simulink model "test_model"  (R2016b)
settings: Solver=VariableStepAuto  StartTime=0.0  StopTime=runtime  RelTol=1e-3
InitFcn:
  | clear mex
  | delete test_model_sfun.mexw64
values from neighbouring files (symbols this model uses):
  Delta_T = cell(1,4)    [modelParameters.m]
  F_D = 0    [modelParameters.m]
  g = 9.81    [modelParameters.m]
  Gamma_H = cell(1,4)    [modelParameters.m]
  have_motor_transient = 1    [modelParameters.m]
  height_controlled_o = (((Rm*If        + (((omega0_o * 2 * Rm * Kv * Kq      * Kd + 1)^2) - 1)/(4* Rm*Kv^2*Kq      * Kd))/Vb)*(Pmax - Pmin) + Pmin)    [modelParameters.m]
  i_0 = cell(1,4)    [modelParameters.m]
  If = 0.3836    [modelParameters.m]
  J = diag([ 0.0130 0.0140 0.0285 ])    [modelParameters.m]
  J_L = m_L/12*diag([y_L^2+z_L^2,x_L^2+z_L^2,x_L^2+y_L^2])    [modelParameters.m]
  J_r = cell(1,4)    [modelParameters.m]
  Jreq = 4.2012e-05    [modelParameters.m]
  Jxx = 0.0130    (= 0.013)    [modelParameters.m]
  Jyy = 0.0140    (= 0.014)    [modelParameters.m]
  Jzz = 0.0285    [modelParameters.m]
  K_d = cell(1,4)    [modelParameters.m]
  K_E = cell(1,4)    [modelParameters.m]
  K_H = cell(1,4)    [modelParameters.m]
  K_Q = cell(1,4)    [modelParameters.m]
  K_T = cell(1,4)    [modelParameters.m]
  K_V = cell(1,4)    [modelParameters.m]
  Kd = 1.4852e-07    [modelParameters.m]
  Ki_mahony = 0.001    [modelParameters.m]
  Kp_mahony = 0.4    [modelParameters.m]
  Kq = 96.3422    [modelParameters.m]
  Kt = 1.2007e-05    [modelParameters.m]
  Kv = 96.3422    [modelParameters.m]
  m = 1.216    [modelParameters.m]
  m_L = 0    [modelParameters.m]
  omega0_o = sqrt((m*g)/(4*Kt))    [modelParameters.m]
  omega1_o = sqrt((m*g)/(4*Kt))    [modelParameters.m]
  omega2_o = sqrt((m*g)/(4*Kt))    [modelParameters.m]
  omega3_o = sqrt((m*g)/(4*Kt))    [modelParameters.m]
  omega_0 = cell(1,4)    [modelParameters.m]
  p0 = 0    [modelParameters.m]
  p_0 = cell(1,4)    [modelParameters.m]
  p_max = cell(1,4)    [modelParameters.m]
  phi0 = 0    [modelParameters.m]
  pitch_o = 0    [modelParameters.m]
  pitchrate_o = 0    [modelParameters.m]
  Pmax = 1    [modelParameters.m]
  Pmin = 0    [modelParameters.m]
  psi0 = 0    [modelParameters.m]
  q0 = 0    [modelParameters.m]
  Q_D = 0    [modelParameters.m]
  r0 = 0    [modelParameters.m]
  R_m = cell(1,4)    [modelParameters.m]
  r_oc = [ 0 ; 0 ; 0 ]    [modelParameters.m]
  r_oL = [0; 0; 0]    [modelParameters.m]
  rhx = 0.16    [modelParameters.m]
  rhy = 0.16    [modelParameters.m]
  rhz = 0.03    [modelParameters.m]
  Rm = 0.235    [modelParameters.m]
  roll_o = 0    [modelParameters.m]
  rollrate_o = 0    [modelParameters.m]
  Tc = 0.04    [modelParameters.m]
  theta0 = 0    [modelParameters.m]
  Tq = 0.005    [modelParameters.m]
  u0 = 0    [modelParameters.m]
  v0 = 0    [modelParameters.m]
  Vb = 11.4    [modelParameters.m]
  w0 = 0    [modelParameters.m]
  x0 = 0    [modelParameters.m]
  x_controlled_o = 0    [modelParameters.m]
  x_o = 0    [modelParameters.m]
  x_vel_o = 0    [modelParameters.m]
  y0 = 0    [modelParameters.m]
  y_controlled_o = 0    [modelParameters.m]
  y_o = 0    [modelParameters.m]
  y_vel_o = 0    [modelParameters.m]
  yaw_controlled_o = 0    [modelParameters.m]
  yaw_o = 0    [modelParameters.m]
  yawrate_o = 0    [modelParameters.m]
  z0 = 0    [modelParameters.m]
  z_o = 0    [modelParameters.m]
  z_vel_o = 0    [modelParameters.m]
undefined symbols (not defined in the file or in its folder): Gamma_Omega, Gamma_T, Ki, Kp, r_h, slope, start, Ts, X0
libraries: simulink x16, Derivative x13, dsparch4 x3, vrlib x2
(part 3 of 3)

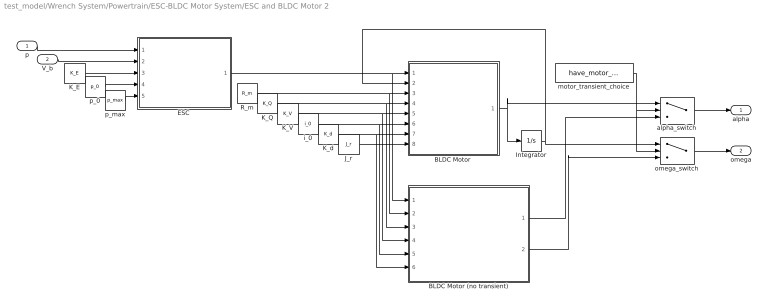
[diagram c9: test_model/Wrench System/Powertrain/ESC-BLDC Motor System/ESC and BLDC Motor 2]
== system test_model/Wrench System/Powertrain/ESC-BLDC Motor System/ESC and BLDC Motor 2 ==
  p : Inport
  V_b : Inport  Port=2
  "BLDC Motor " : MATLAB Function  TreatAsAtomicUnit=on
  BLDC Motor (no transient) : MATLAB Function  TreatAsAtomicUnit=on
  "ESC " : MATLAB Function  TreatAsAtomicUnit=on
  Integrator : Integrator  InitialCondition=omega_0  ContinuousStateAttributes='omega'
  J_r : Constant  Value=J_r
  K_E : Constant  Value=K_E
  K_Q : Constant  Value=K_Q
  K_V : Constant  Value=K_V
  K_d : Constant  Value=K_d
  R_m : Constant  Value=R_m
  alpha_switch : Switch  Criteria=u2 ~= 0
  i_0 : Constant  Value=i_0
  motor_transient_choice : Constant  Value=have_motor_transient
  omega_switch : Switch  Criteria=u2 ~= 0
  p_0 : Constant  Value=p_0
  p_max : Constant  Value=p_max
  alpha : Outport
  omega : Outport  Port=2
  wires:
  motor_transient_choice/1 -> omega_switch/2, alpha_switch/2
  omega_switch/1 -> omega/1
  alpha_switch/1 -> alpha/1
  BLDC Motor (no transient)/2(omega) -> omega_switch/3
  BLDC Motor (no transient)/1(alpha) -> alpha_switch/3
  Integrator/1 -> omega_switch/1, "BLDC Motor "/2(omega)
  "ESC "/1(V) -> BLDC Motor (no transient)/1(V), "BLDC Motor "/1(V)
  p/1 -> "ESC "/1(p)
  V_b/1 -> "ESC "/2(V_b)
  K_E/1 -> "ESC "/3(K_E)
  p_0/1 -> "ESC "/4(p_0)
  p_max/1 -> "ESC "/5(p_max)
  J_r/1 -> "BLDC Motor "/8(J_r)
  R_m/1 -> BLDC Motor (no transient)/2(R_m), "BLDC Motor "/3(R_m)
  "BLDC Motor "/1(alpha) -> alpha_switch/1, Integrator/1
  K_Q/1 -> BLDC Motor (no transient)/3(K_Q), "BLDC Motor "/4(K_Q)
  K_V/1 -> BLDC Motor (no transient)/4(K_V), "BLDC Motor "/5(K_V)
  i_0/1 -> BLDC Motor (no transient)/5(i_0), "BLDC Motor "/6(i_0)
  K_d/1 -> BLDC Motor (no transient)/6(K_d), "BLDC Motor "/7(K_d)

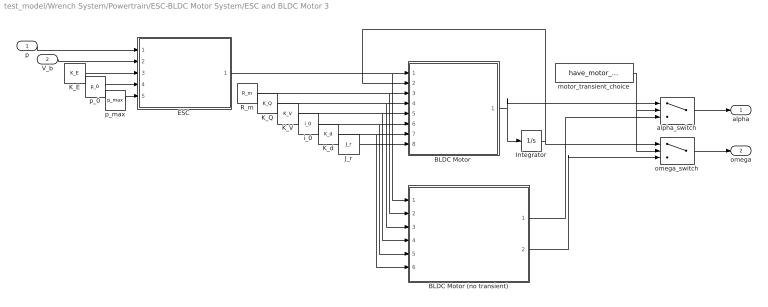
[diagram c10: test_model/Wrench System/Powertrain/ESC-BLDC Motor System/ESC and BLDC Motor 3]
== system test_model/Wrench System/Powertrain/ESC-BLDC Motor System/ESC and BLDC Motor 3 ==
  p : Inport
  V_b : Inport  Port=2
  "BLDC Motor " : MATLAB Function  TreatAsAtomicUnit=on
  BLDC Motor (no transient) : MATLAB Function  TreatAsAtomicUnit=on
  "ESC " : MATLAB Function  TreatAsAtomicUnit=on
  Integrator : Integrator  InitialCondition=omega_0  ContinuousStateAttributes='omega'
  J_r : Constant  Value=J_r
  K_E : Constant  Value=K_E
  K_Q : Constant  Value=K_Q
  K_V : Constant  Value=K_V
  K_d : Constant  Value=K_d
  R_m : Constant  Value=R_m
  alpha_switch : Switch  Criteria=u2 ~= 0
  i_0 : Constant  Value=i_0
  motor_transient_choice : Constant  Value=have_motor_transient
  omega_switch : Switch  Criteria=u2 ~= 0
  p_0 : Constant  Value=p_0
  p_max : Constant  Value=p_max
  alpha : Outport
  omega : Outport  Port=2
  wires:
  motor_transient_choice/1 -> omega_switch/2, alpha_switch/2
  omega_switch/1 -> omega/1
  alpha_switch/1 -> alpha/1
  BLDC Motor (no transient)/2(omega) -> omega_switch/3
  BLDC Motor (no transient)/1(alpha) -> alpha_switch/3
  Integrator/1 -> omega_switch/1, "BLDC Motor "/2(omega)
  "ESC "/1(V) -> BLDC Motor (no transient)/1(V), "BLDC Motor "/1(V)
  p/1 -> "ESC "/1(p)
  V_b/1 -> "ESC "/2(V_b)
  K_E/1 -> "ESC "/3(K_E)
  p_0/1 -> "ESC "/4(p_0)
  p_max/1 -> "ESC "/5(p_max)
  J_r/1 -> "BLDC Motor "/8(J_r)
  R_m/1 -> BLDC Motor (no transient)/2(R_m), "BLDC Motor "/3(R_m)
  "BLDC Motor "/1(alpha) -> alpha_switch/1, Integrator/1
  K_Q/1 -> BLDC Motor (no transient)/3(K_Q), "BLDC Motor "/4(K_Q)
  K_V/1 -> BLDC Motor (no transient)/4(K_V), "BLDC Motor "/5(K_V)
  i_0/1 -> BLDC Motor (no transient)/5(i_0), "BLDC Motor "/6(i_0)
  K_d/1 -> BLDC Motor (no transient)/6(K_d), "BLDC Motor "/7(K_d)

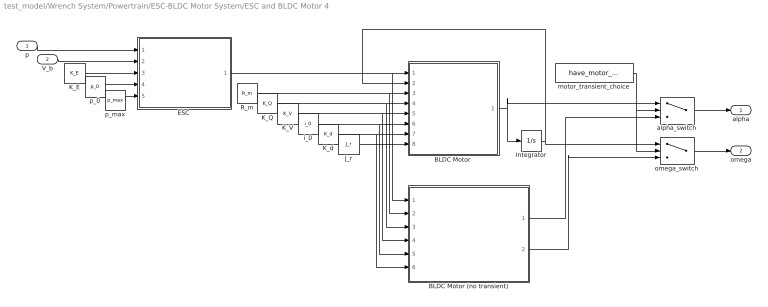
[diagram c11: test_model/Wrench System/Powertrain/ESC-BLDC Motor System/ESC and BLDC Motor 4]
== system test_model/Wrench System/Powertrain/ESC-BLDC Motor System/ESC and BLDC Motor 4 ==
  p : Inport
  V_b : Inport  Port=2
  "BLDC Motor " : MATLAB Function  TreatAsAtomicUnit=on
  BLDC Motor (no transient) : MATLAB Function  TreatAsAtomicUnit=on
  "ESC " : MATLAB Function  TreatAsAtomicUnit=on
  Integrator : Integrator  InitialCondition=omega_0  ContinuousStateAttributes='omega'
  J_r : Constant  Value=J_r
  K_E : Constant  Value=K_E
  K_Q : Constant  Value=K_Q
  K_V : Constant  Value=K_V
  K_d : Constant  Value=K_d
  R_m : Constant  Value=R_m
  alpha_switch : Switch  Criteria=u2 ~= 0
  i_0 : Constant  Value=i_0
  motor_transient_choice : Constant  Value=have_motor_transient
  omega_switch : Switch  Criteria=u2 ~= 0
  p_0 : Constant  Value=p_0
  p_max : Constant  Value=p_max
  alpha : Outport
  omega : Outport  Port=2
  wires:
  motor_transient_choice/1 -> omega_switch/2, alpha_switch/2
  omega_switch/1 -> omega/1
  alpha_switch/1 -> alpha/1
  BLDC Motor (no transient)/2(omega) -> omega_switch/3
  BLDC Motor (no transient)/1(alpha) -> alpha_switch/3
  Integrator/1 -> omega_switch/1, "BLDC Motor "/2(omega)
  "ESC "/1(V) -> BLDC Motor (no transient)/1(V), "BLDC Motor "/1(V)
  p/1 -> "ESC "/1(p)
  V_b/1 -> "ESC "/2(V_b)
  K_E/1 -> "ESC "/3(K_E)
  p_0/1 -> "ESC "/4(p_0)
  p_max/1 -> "ESC "/5(p_max)
  J_r/1 -> "BLDC Motor "/8(J_r)
  R_m/1 -> BLDC Motor (no transient)/2(R_m), "BLDC Motor "/3(R_m)
  "BLDC Motor "/1(alpha) -> alpha_switch/1, Integrator/1
  K_Q/1 -> BLDC Motor (no transient)/3(K_Q), "BLDC Motor "/4(K_Q)
  K_V/1 -> BLDC Motor (no transient)/4(K_V), "BLDC Motor "/5(K_V)
  i_0/1 -> BLDC Motor (no transient)/5(i_0), "BLDC Motor "/6(i_0)
  K_d/1 -> BLDC Motor (no transient)/6(K_d), "BLDC Motor "/7(K_d)

== matlab function test_model/Actuation/Gravity

 ==
function E_Fg = gravity(m, g)

E_Fg = [0; 0; m*g];

== matlab function test_model/Actuation/Lbe





 ==
function E_ro  = linear_body_earth_conversion(B_vo, euler_angles)

euler_rates = zeros(3,1);
E_ro = zeros(3,1);

phi = euler_angles(1);
theta = euler_angles(2);
psi = euler_angles(3);

Leb = [cos(theta)*cos(psi), sin(phi)*sin(theta)*cos(psi)-cos(phi)*sin(psi), cos(phi)*sin(theta)*cos(psi)+sin(phi)*sin(psi); ...
       cos(theta)*sin(psi), sin(phi)*sin(theta)*sin(psi)+cos(phi)*cos(psi), cos(phi)*sin(theta)*sin(psi)-sin(phi)*cos(psi); ...
           -sin(theta)    ,                sin(phi)*cos(theta)            ,                 cos(phi)*cos(theta)           ];

E_ro = Leb * B_vo;

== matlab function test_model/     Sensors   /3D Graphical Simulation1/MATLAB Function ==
function y = eigenaxis_ucart(u)


if abs(u(1))< 0.0001
    u(1) = 0.0001;
end

if abs(u(2))< 0.0001
    u(2) = 0.0001;
end

if abs(u(3))< 0.0001
    u(3) = 0.0001;
end

u = [ -u(1); -u(2); u(3) ];% [Pitch, Yaw, Roll] 

C11 = cos(u(2))*cos(u(3));
C12 = cos(u(2))*sin(u(3));
C13 = -sin(u(2));
C21 = sin(u(1))*sin(u(2))*cos(u(3))-cos(u(1))*sin(u(3));
C22 = sin(u(1))*sin(u(2))*sin(u(3))+cos(u(1))*cos(u(3));
C23 = sin(u(1))*cos(u(2));
C31 = cos(u(1))*sin(u(2))*cos(u(3))+sin(u(1))*sin(u(3));
C32 = cos(u(1))*sin(u(2))*sin(u(3))-sin(u(1))*cos(u(3));
C33 = cos(u(1))*cos(u(2));
    
theta = acos(0.5*(C11+C22+C33-1));

e = [C23-C32; C31-C13; C12-C21]/(2*sin(theta));
    
y = [e; theta];

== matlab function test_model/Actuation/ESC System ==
function Vb_eff   = ESC(P, Pmin, Pmax, Vb)

P1 = P(1);
P2 = P(2);
P3 = P(3);
P4 = P(4);

% Define u_Pi for each of the rotors, limiting it to be greater than 0
u_P0 = (P1 - Pmin) / (Pmax - Pmin);
u_P1 = (P2 - Pmin) / (Pmax - Pmin);
u_P2 = (P3 - Pmin) / (Pmax - Pmin);
u_P3 = (P4 - Pmin) / (Pmax - Pmin);


% Determine the effective battery voltage from each ESC
Vb_eff_0 = u_P0 * Vb;
Vb_eff_1 = u_P1 * Vb;
Vb_eff_2 = u_P2 * Vb;
Vb_eff_3 = u_P3 * Vb;
    
Vb_eff = [Vb_eff_0, Vb_eff_1, Vb_eff_2, Vb_eff_3];

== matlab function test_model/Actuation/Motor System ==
function w_dot = motor(Vb_eff, w, Rm, Kv, Kq, Kd, If, Jreq)

% Define each motors effective battery voltage
Vb_eff_0 = Vb_eff(1);
Vb_eff_1 = Vb_eff(2);
Vb_eff_2 = Vb_eff(3);
Vb_eff_3 = Vb_eff(4);

% Determine the angular velocity of each rotor from feedback
w_0 = w(1);
w_1 = w(2);
w_2 = w(3);
w_3 = w(4);

% Determine angular acceleration of each rotor
w_0_dot = 1/(Jreq*Rm*Kq) * Vb_eff_0 - 1/(Jreq*Rm*Kq*Kv) * w_0 - 1/(Jreq*Kq)*If - (Kd/Jreq) * w_0^2;
w_1_dot = 1/(Jreq*Rm*Kq) * Vb_eff_1 - 1/(Jreq*Rm*Kq*Kv) * w_1 - 1/(Jreq*Kq)*If - (Kd/Jreq) * w_1^2;
w_2_dot = 1/(Jreq*Rm*Kq) * Vb_eff_2 - 1/(Jreq*Rm*Kq*Kv) * w_2 - 1/(Jreq*Kq)*If - (Kd/Jreq) * w_2^2;
w_3_dot = 1/(Jreq*Rm*Kq) * Vb_eff_3 - 1/(Jreq*Rm*Kq*Kv) * w_3 - 1/(Jreq*Kq)*If - (Kd/Jreq) * w_3^2;

w_dot = [w_0_dot, w_1_dot, w_2_dot, w_3_dot];

== matlab function test_model/Actuation/Rotor System







 ==
function [B_omega_dot, B_vo_dot]= rotor(w_dot, w, B_Fg, B_omega, B_vo, m, Kt, Kd, rhx, rhy, rhz, Jreq, Jxx, Jyy, Jzz, r_oc)

% Create J vector
J = [Jxx,  0 ,  0 ; ...
      0 , Jyy,  0 ; ...
      0 ,  0 , Jzz;];
  
r_oc_X = [0, -r_oc(3), r_oc(2); r_oc(3), 0, -r_oc(1); -r_oc(2), r_oc(1), 0];

% Create r_hi vector
rh_0 = [-rhx; rhy; -rhz];
rh_1 = [rhx; rhy; -rhz];
rh_2 = [-rhx; -rhy; -rhz];
rh_3 = [rhx; -rhy; -rhz];

% Define 3x3 Identity Matrix
I = eye(3);

% Create gamma vectors
gamma_Ti = [0; 0; -1];
gamma_omega_03 = [0; 0; 1];  %Rotors 0 and 3 use this gamma_omega vector
gamma_omega_12 = [0; 0; -1]; %Rotors 1 and 2 use this gamma_omega vector

% Define angular velocities for each rotor
w_0 = w(1);
w_1 = w(2);
w_2 = w(3);
w_3 = w(4);

% Define angular acceleration for each rotor
w_0_dot = w_dot(1);
w_1_dot = w_dot(2);
w_2_dot = w_dot(3);
w_3_dot = w_dot(4);

% Define the rotor force in the z-direction from each rotor
B_Fr_0 = Kt * w_0 * w_0 * gamma_Ti;
B_Fr_1 = Kt * w_1 * w_1 * gamma_Ti;
B_Fr_2 = Kt * w_2 * w_2 * gamma_Ti;
B_Fr_3 = Kt * w_3 * w_3 * gamma_Ti;

% Sum up the rotor forces in the z-direction from each vector to get the
% total body force in the z-direction
B_Fr = B_Fr_0 + B_Fr_1 + B_Fr_2 + B_Fr_3;

% Define the in-plane drag and induced torque produced by each rotor
 B_Q_d0 = -1 * Kd * w_0 * w_0 * gamma_omega_03;
 B_Q_d1 = -1 * Kd * w_1 * w_1 * gamma_omega_12;
 B_Q_d2 = -1 * Kd * w_2 * w_2 * gamma_omega_12;
 B_Q_d3 = -1 * Kd * w_3 * w_3 * gamma_omega_03;

% Sum up the total in-plane drag and induced torque to get the total
% in-plane drag and induced torque on the body
B_Q_d = B_Q_d0 + B_Q_d1 + B_Q_d2 + B_Q_d3;

% Define the force lever arm torque created from the force produced by each
% rotor in the z-direction
B_Q_F0 = cross( rh_0, B_Fr_0 );
B_Q_F1 = cross( rh_1, B_Fr_1 );
B_Q_F2 = cross( rh_2, B_Fr_2 );
B_Q_F3 = cross( rh_3, B_Fr_3 );

B_Q_F = B_Q_F0 + B_Q_F1 + B_Q_F2 + B_Q_F3;

%Define the change in angular momentum torque produced by each rotor 
B_Q_L0 = -1 * Jreq * ( cross(B_omega, w_0 * gamma_omega_03) + w_0_dot * gamma_omega_03 );
B_Q_L1 = -1 * Jreq * ( cross(B_omega, w_1 * gamma_omega_12) + w_1_dot * gamma_omega_12 ); 
B_Q_L2 = -1 * Jreq * ( cross(B_omega, w_2 * gamma_omega_12) + w_2_dot * gamma_omega_12 ); 
B_Q_L3 = -1 * Jreq * ( cross(B_omega, w_3 * gamma_omega_03) + w_3_dot * gamma_omega_03 );

% Sum up the total change in angular momentum torque produced by each rotor
B_Q_L = B_Q_L0 + B_Q_L1 + B_Q_L2 + B_Q_L3;

% Define the total rotor system torque as the sum of the in-plane drag and
% induced torque, force lever arm torque, and change in angular momentum
% torques
B_Q = B_Q_d + B_Q_F + B_Q_L;

% Define the body forces in the z-direction from each vector to get the
% total body force in the z-direction
B_F = B_Fr + B_Fg; 

% Determine the dynamics of the system
M = [m * I , -m * r_oc_X; 
    zeros(3,3), J];

dynamics = M^(-1) *     [B_F - cross( B_omega, m*(B_vo + cross(B_omega, r_oc))); ...
     B_Q - cross(B_omega, J * B_omega) - cross(r_oc, B_F)];

% Define the body frame angular velocities
B_vo_dot = dynamics(1:3);

% Define the body frame linear velocities
B_omega_dot = dynamics(4:6);
 
% B_vo_dot = (m*I)^(-1) * ( B_F - cross( B_omega, m*(B_vo + cross(B_omega, r_oc)) ) );
% B_omega_dot = J ^(-1) * ( B_Q - cross(B_omega, J * B_omega) - cross(r_oc, B_F)  );

== matlab function test_model/Actuation/Aeb














 ==
function euler_rates = angular_body_earth_conversion(B_omega, euler_angles)

phi = euler_angles(1);
theta = euler_angles(2);

Aeb = [1,  sin(phi)*tan(theta), cos(phi)*tan(theta); ...
       0,      cos(phi)       ,        -sin(phi)   ; ...
       0,  sin(phi)/cos(theta), cos(phi)/cos(theta)];

   
euler_rates = Aeb * B_omega;

== matlab function test_model/Actuation/Lbe

















 ==
function [B_Fg, B_g]  = linear_earth_body_conversion(E_Fg, euler_angles, m)

phi = euler_angles(1);
theta = euler_angles(2);
psi = euler_angles(3);

Lbe = [             cos(theta)*cos(psi)              ,          cos(theta)*sin(psi)                  ,     -sin(theta)    ; ...
       sin(phi)*sin(theta)*cos(psi)-cos(phi)*sin(psi), sin(phi)*sin(theta)*sin(psi)+cos(phi)*cos(psi), sin(phi)*cos(theta); ...
       cos(phi)*sin(theta)*cos(psi)+sin(phi)*sin(psi), cos(phi)*sin(theta)*sin(psi)-sin(phi)*cos(psi), cos(phi)*cos(theta)];

B_Fg = Lbe * E_Fg;

B_g = B_Fg/m;

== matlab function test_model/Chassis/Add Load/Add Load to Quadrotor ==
function [m,J,r_oc] = add_load(m_0,J_0,r_oc_0,m_l,J_l,r_ol)
%#codegen
r_oc = (m_0*r_oc_0 + m_l*r_ol)/(m_0+m_l); 
m = m_0 + m_l; 
r_cl = -r_oc + r_ol; 
r_co = -r_oc; 
J = J_0 + J_l + m_0*(r_co'*r_co*eye(3) - r_co*r_co') + m_l*(r_cl'*r_cl*eye(3) - r_cl*r_cl'); 

end

== matlab function test_model/     Sensors   /IMU





/






 ==
function [accelReading,gyroReading] = idealIMU(B_vo_dot, B_vo, B_Omega, B_g, g, r_oc)
%#codegen

a = B_vo_dot + cross(B_Omega,B_vo); % body frame acceleration 

accelReading = (a - B_g)/g ; % accelerometer reading (ideal)

gyroReading = B_Omega ; % gyroscope reading (ideal) 

end

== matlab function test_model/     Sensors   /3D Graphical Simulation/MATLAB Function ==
function y = eigenaxis_ucart(u)


if abs(u(1))< 0.0001
    u(1) = 0.0001;
end

if abs(u(2))< 0.0001
    u(2) = 0.0001;
end

if abs(u(3))< 0.0001
    u(3) = 0.0001;
end

u = [ -u(1); -u(2); u(3) ];% [Pitch, Yaw, Roll] 

C11 = cos(u(2))*cos(u(3));
C12 = cos(u(2))*sin(u(3));
C13 = -sin(u(2));
C21 = sin(u(1))*sin(u(2))*cos(u(3))-cos(u(1))*sin(u(3));
C22 = sin(u(1))*sin(u(2))*sin(u(3))+cos(u(1))*cos(u(3));
C23 = sin(u(1))*cos(u(2));
C31 = cos(u(1))*sin(u(2))*cos(u(3))+sin(u(1))*sin(u(3));
C32 = cos(u(1))*sin(u(2))*sin(u(3))-sin(u(1))*cos(u(3));
C33 = cos(u(1))*cos(u(2));
    
theta = acos(0.5*(C11+C22+C33-1));

e = [C23-C32; C31-C13; C12-C21]/(2*sin(theta));
    
y = [e; theta];

== matlab function test_model/     Sensors   /Aeb









 ==
function euler_rates_IMU = angular_body_earth_conversion(gyro_reading, euler_angles_filtered)

phi = euler_angles_filtered(1);
theta = euler_angles_filtered(2);

Aeb = [1, sin(phi)*tan(theta), cos(phi)*tan(theta); ...
       0,     cos(phi)       ,        -sin(phi)   ; ...
       0,  sin(phi)/cos(theta), cos(phi)/cos(theta)];

   
euler_rates_IMU = Aeb * gyro_reading;

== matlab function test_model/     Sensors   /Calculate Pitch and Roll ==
function [accel_pitch, accel_roll] = getPitchAndRoll(accel_reading)

x_accel = accel_reading(1);
y_accel = accel_reading(2);
z_accel = accel_reading(3);

accel_pitch = atan(x_accel/sqrt(y_accel^2 + z_accel^2));
accel_roll = atan( -y_accel/( sqrt(z_accel^2 + x_accel^2))  );

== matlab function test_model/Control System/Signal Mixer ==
function P  = signal_mixer(height_controlled, y_controlled, x_controlled, yaw_controlled)

controller_outputs = [ height_controlled; x_controlled; y_controlled; yaw_controlled ];
signal_mixer = [ 1, -1, -1, -1; ... 
                 1,  1, -1,  1; ...
                 1, -1,  1,  1; ...
                 1,  1,  1, -1 ];
             
P = signal_mixer * controller_outputs;

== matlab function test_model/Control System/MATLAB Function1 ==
function [z_corr, y_cor, x_corr, yaw_corr, pid_y_out, pid_roll_out] = c_controller(set_x, set_y, set_z, set_yaw, ...
    cur_x, cur_y, cur_z, ...
    cur_phi, cur_theta, cur_psi, ...
    cur_phi_d, cur_theta_d, cur_psi_d, vrpn_id, Tc)

out_z = -1;
out_y = -1;
out_x = -1;
out_yaw = -1;
c_pid_y = -1;
c_pid_roll = -1;

coder.ceval('c_controller', vrpn_id, Tc, set_x, set_y, set_z, set_yaw, ...
                    cur_x, cur_y, cur_z, ...
                    cur_phi, cur_theta, cur_psi, ...
                    cur_phi_d, cur_theta_d, cur_psi_d, ...
                    coder.wref(out_z), coder.wref(out_y), coder.wref(out_x), coder.wref(out_yaw), ...
                    coder.wref(c_pid_y), coder.wref(c_pid_roll));

z_corr = out_z;
y_cor = out_y;
x_corr = out_x;
pid_y_out = c_pid_y;
pid_roll_out = c_pid_roll;
yaw_corr = out_yaw;

== matlab function test_model/     Sensors   /Aeb_c









1 ==
function euler_rates_IMU = angular_body_earth_conversion(gyro_reading, euler_angles_filtered)

phi = euler_angles_filtered(1);
theta = euler_angles_filtered(2);
psi = NaN;

phi_dot = -1;
theta_dot = -1;
psi_dot = -1;

p = gyro_reading(1);
q = gyro_reading(2);
r = gyro_reading(3);

coder.ceval( 'aeb_mat', p, q, r, phi, theta, psi, coder.wref(phi_dot), ...
    coder.wref(theta_dot), coder.wref(psi_dot) );

   
euler_rates_IMU = [phi_dot; theta_dot; psi_dot];

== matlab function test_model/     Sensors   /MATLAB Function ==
function euler_angles_IMU  = complimentaryFilterC(accel_pitch, accel_roll, euler_rates_gyro)

euler_x = euler_rates_gyro(1);
euler_y = euler_rates_gyro(2);

filtered_pitch = -1;
filtered_roll = -1;

coder.ceval('compl_filter', accel_pitch, accel_roll, euler_x, euler_y, ...
            coder.wref(filtered_pitch), coder.wref(filtered_roll));

euler_angles_IMU = [filtered_roll; filtered_pitch];

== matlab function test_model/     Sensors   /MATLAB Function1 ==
function [accel_pitch, accel_roll]  = angle_IMU_C(accel_reading)

accel_x = accel_reading(1);
accel_y = accel_reading(2);
accel_z = accel_reading(3);

calculated_pitch = -1;
calculated_roll = -1;

coder.ceval('angle_accel', accel_x, accel_y, accel_z, coder.wref(calculated_pitch), coder.wref(calculated_roll));

accel_pitch = calculated_pitch;
accel_roll = calculated_roll;

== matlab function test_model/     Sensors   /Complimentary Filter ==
function euler_angles_IMU   = complimentaryFilter(accel_pitch, accel_roll, euler_rates_gyro, prev_euler_angles)

k_gyro = 0.99; 
k_accel = 1-k_gyro; 

Ts = 0.005; % 5 milliseconds

prev_phi = prev_euler_angles(1);
prev_theta = prev_euler_angles(2);

prev_phi_dot = euler_rates_gyro(1);
prev_theta_dot = euler_rates_gyro(2);

integrated_phi_gyro = Ts * prev_phi_dot + prev_phi;
integrated_theta_gyro = Ts * prev_theta_dot + prev_theta;

phi = k_gyro * integrated_phi_gyro + k_accel * accel_roll;
theta = k_gyro * integrated_theta_gyro + k_accel * accel_pitch;

euler_angles_IMU = [phi; theta];

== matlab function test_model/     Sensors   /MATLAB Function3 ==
function [eulerAngles, integralFeedback, quaternions] = ...
    mahonyFilter(accelReadings, gyroReadings, quaternions_prev, ...
    integralFeedback_prev, Tq, Kp_mahony, Ki_mahony)
%     mahonyFilter(accelReadings, gyroReadings, eulerAngles_prev, ...
%     integralFeedback_prev, Tq, Kp_mahony, Ki_mahony)
    
    
    %Save quadcopter loop time as dt
    dt = Tq;

    %Pull accelerometer readings and negate them to compare
    accel_x = accelReadings(1);
    accel_y = accelReadings(2);
    accel_z = accelReadings(3);
    
    %Negate the accelerometer values to compare with direction of the
    %gravity vector
    accel_x = (-1) * accel_x;
    accel_y = (-1) * accel_y;
    accel_z = (-1) * accel_z;

    %Pull gyroscope readings
    gyro_x = gyroReadings(1);
    gyro_y = gyroReadings(2);
    gyro_z = gyroReadings(3);

    %Pull previous Euler angles
%     roll_prev = eulerAngles_prev(1);
%     pitch_prev = eulerAngles_prev(2);
%     yaw_prev = eulerAngles_prev(3);
    
    %Pull previous integral feedback terms
    integralFeedback_x_prev = integralFeedback_prev(1);
    integralFeedback_y_prev = integralFeedback_prev(2);
    integralFeedback_z_prev = integralFeedback_prev(3);

    %Calculate half cosines and sines for the quaternion elements
%     cosHalfRoll = cos( 0.5 * roll_prev );
%     sinHalfRoll = sin( 0.5 * roll_prev );
%     cosHalfPitch = cos( 0.5 * pitch_prev );
%     sinHalfPitch = sin( 0.5 * pitch_prev );
%     cosHalfYaw = cos( 0.5 * yaw_prev );
%     sinHalfYaw = sin( 0.5 * yaw_prev );

    %Calculate the quaternion elements
%     q0 = cosHalfRoll * cosHalfPitch * cosHalfYaw + ...
%         sinHalfRoll * sinHalfPitch * sinHalfYaw;
% 
%     q1 = sinHalfRoll * cosHalfPitch * cosHalfYaw - ...
%         cosHalfRoll * sinHalfPitch * sinHalfYaw;
% 
%     q2 = cosHalfRoll * sinHalfPitch * cosHalfYaw + ...
%         sinHalfRoll * cosHalfPitch * sinHalfYaw;
% 
%     q3 = (-1) * sinHalfRoll * sinHalfPitch * cosHalfYaw + ...
%         cosHalfRoll * cosHalfPitch * sinHalfYaw;

    %Pull the quaternion values
    q0 = quaternions_prev(1);
    q1 = quaternions_prev(2);
    q2 = quaternions_prev(3);
    q3 = quaternions_prev(4);


    %Calculate the rate of change of the quaternion from the gyroscope
%     q0_dot = 0.5 * ( (-1)*(q1 * gyro_x) - (q2 * gyro_y) - (q3 * gyro_z) );
%     q1_dot = 0.5 * ( (q0 * gyro_x) + (q2 * gryo_z) - (q3 * gyro_y) );
%     q2_dot = 0.5 * ( (q0 * gyro_y) - (q1 * gyro_z) + (q3 * gyro_x) );
%     q3_dot = 0.5 * ( (q0 * gyro_z) + (q1 * gyro_y) - (q2 * gyro_x) );

    %Define initial values for the corrected gyroscope values
    gyro_x_corrected = gyro_x;
    gyro_y_corrected = gyro_y;
    gyro_z_corrected = gyro_z;
    
    %Define initial values for the corrected integral feedback values
    integralFeedback_x = integralFeedback_x_prev;
    integralFeedback_y = integralFeedback_y_prev;
    integralFeedback_z = integralFeedback_z_prev;

    %Only compute the feedback if the accelerometer measurements are valid
    %This prevents NaN values when normalizing the accelerometer measurements
    if( accel_x ~= 0 && accel_y ~= 0  && accel_z ~= 0 )

       %Check... maybe we don't need to do this normalization...
       %Ideally our accelerometer readings should have a magnitude of 1, but
       %this is usually not the case with data we have collected
       accel_mag = ( (accel_x ^ 2) + (accel_y ^ 2) + (accel_z ^ 2) ) ^ 0.5;
       accel_x = accel_x / accel_mag;
       accel_y = accel_y / accel_mag;
       accel_z = accel_z / accel_mag;

       %Estimate direction of gravity
       vx = 2 * ( (q1 * q3) - (q0 * q2) );
       vy = 2 * ( (q0 * q1) + (q2 * q3) );
       vz = (2 * q0 * q0) - (q3 * q3);
       
       %Error is the sum of the cross product between the estimated and
       %measured direction of gravity
       ex = (accel_y * vz) - (accel_z * vy);
       ey = (accel_z * vx) - (accel_x * vz);
       ez = (accel_x * vy) - (accel_y * vx);
       
       %Compute and apply the proportional feedback
       gyro_x_corrected = gyro_x + (Kp_mahony * ex);
       gyro_y_corrected = gyro_y + (Kp_mahony * ey);
       gyro_z_corrected = gyro_z + (Kp_mahony * ez);

       %Compute and apply the integral feedback, if it is enabled
       if ( Ki_mahony > 0 )
           
           %Integrate digitally based on sample time and scale by Ki, and
           %accumulate the integral term by adding this to the previous
           %feedback term
           integralFeedback_x = (Ki_mahony * ex * dt) + ...
               integralFeedback_x_prev;
           integralFeedback_y = (Ki_mahony * ey * dt) + ...
               integralFeedback_y_prev;
           integralFeedback_z = (Ki_mahony * ez * dt) + ...
               integralFeedback_z_prev;
           
           %Correct the gyroscope values using the new integral feedback
           gyro_x_corrected = gyro_x_corrected + integralFeedback_x;
           gyro_y_corrected = gyro_y_corrected + integralFeedback_y;
           gyro_z_corrected = gyro_z_corrected + integralFeedback_z;
           
       else
           
           %Otherwise, reset the integral terms to zero to prevent windup
           integralFeedback_x = 0;
           integralFeedback_y = 0;
           integralFeedback_z = 0;
           
       end %if ( Ki_mahoney > 0 )

    end %if ( accel_x ~= 0 && accel_y ~= 0 && accel_z ~= 0 )

    %Integrate the rate of change of the quaternion
    %First, pre-multiply the common factors to the gyro reading values
    gyro_x_corrected = gyro_x_corrected * (0.5 * dt);
    gyro_y_corrected = gyro_y_corrected * (0.5 * dt);
    gyro_z_corrected = gyro_z_corrected * (0.5 * dt);
    
    %Now, create temporary variales for the first three quaternion values
    qa = q0;
    qb = q1;
    qc = q2;
    
    %Now perform calculation to integrate the rate of the quaternion
    q0 = q0 - (qb * gyro_x_corrected) - (qc * gyro_y_corrected) - ...
        (q3 * gyro_z_corrected);
    q1 = q1 + (qa * gyro_x_corrected) + (qc * gyro_z_corrected) - ...
        (q3 * gyro_y_corrected);
    q2 = q2 + (qa * gyro_y_corrected) - (qb * gyro_z_corrected) + ...
        (q3 * gyro_x_corrected);
    q3 = q3 + (qa * gyro_z_corrected) + (qb * gyro_y_corrected) - ...
        (qc * gyro_x_corrected);
    
    %Normalize quaternion
    quaternion_mag = ( (q0 * q0) + (q1 * q1) + (q2 * q2) + (q3 * q3) ) ^ 0.5;
    q0 = q0 / quaternion_mag;
    q1 = q1 / quaternion_mag;
    q2 = q2 / quaternion_mag;
    q3 = q3 / quaternion_mag;
    
    %Estimate the gravity direction from the quaternion values
    grav_x = 2 * ( (q1 * q3) - (q0 * q2) );
    grav_y = 2 * ( (q0 * q1) + (q2 * q3) );
    grav_z = (q0 * q0) - (q1 * q1) - (q2 * q2) + (q3 * q3);
    
    %Limit the gravity vector in x-direction to maintain a magnitude of 1
%     grav_x = min( grav_x , 1 );
%     grav_x = max( grav_x , -1 );

    %Normalize the gravity vector
    grav_mag = sqrt( ( grav_x * grav_x ) + ( grav_y * grav_y ) + ...
        ( grav_z * grav_z ) );
    grav_x = grav_x / grav_mag;
    grav_y = grav_y / grav_mag;
    grav_z = grav_z / grav_mag;
    
    %Calculate the pitch, roll, and yaw
    yaw = atan2( 2 * ( (q0 * q3) + (q1 * q2) ) , ...
        (q0 * q0) + (q1 * q1) - (q2 * q2) - (q3 * q3) );
    pitch = asin( (-1) * grav_x );
    roll = atan2( grav_y , grav_z );
    
    %Create a vector of current integral feedback terms to output
    integralFeedback = [ integralFeedback_x ; ...
        integralFeedback_y ; integralFeedback_z ];
    
    %Create a vector of the corrected gyroscope terms
    %gyroReadings_corrected = [ gyro_x_corrected ; ...
    %    gyro_y_corrected ; gyro_z_corrected ];
    
    %Create a vector of the newly calculated quaternion values
    quaternions = [ q0 ; q1 ; q2 ; q3 ];
    
    %Create a vector of the calculated Euler angles
    eulerAngles = [ roll ;  pitch ; yaw ];
    
end %function

== matlab function test_model/Chassis/Body Frame 
Angular Velocity 
to Euler Rates ==
function dot_Theta = pqr2euler(Omega_B,Theta)
%#codegen

phi = Theta(1); 
theta = Theta(2); 
%psi = Theta(3); 

A_BE = [ 1 sin(phi)*tan(theta) cos(phi)*tan(theta); 
         0      cos(phi)            -sin(phi)     ; 
         0 sin(phi)/cos(theta) cos(phi)/cos(theta) ];
     
dot_Theta = A_BE*Omega_B; 

end

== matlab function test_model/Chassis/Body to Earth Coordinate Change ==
function x_E = body2earth(x_B,Theta)
%#codegen

phi = Theta(1); 
theta = Theta(2); 
psi = Theta(3); 

L_BE = [ cos(theta)*cos(psi) , sin(phi)*sin(theta)*cos(psi)-cos(phi)*sin(psi) , cos(phi)*sin(theta)*cos(psi)+sin(phi)*sin(psi) ; 
         cos(theta)*sin(psi) , sin(phi)*sin(theta)*sin(psi)+cos(phi)*cos(psi) , cos(phi)*sin(theta)*sin(psi)-sin(phi)*cos(psi) ; 
                 -sin(theta) ,                            sin(phi)*cos(theta) , cos(phi)*cos(theta) ];
x_E = L_BE*x_B; 

end

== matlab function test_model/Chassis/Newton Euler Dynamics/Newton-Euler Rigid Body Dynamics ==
function [dv,dOmega] = newton_euler(F,Q,v,Omega,m,J,r_oc)
%#codegen 

r_oc_X = [ 0 -r_oc(3) r_oc(2) ; r_oc(3) 0 -r_oc(1) ; -r_oc(2) r_oc(1) 0 ]; 

M = [ m*eye(3) , -m*r_oc_X ; 
    zeros(3,3) , J ];

f = M^-1*[F - m*cross(Omega,v) - m*cross(Omega,cross(Omega,r_oc)) ; ... 
          Q - cross(Omega,J*Omega) - cross(r_oc,F) ];

dv = f(1:3); 
dOmega = f(4:6); 

end

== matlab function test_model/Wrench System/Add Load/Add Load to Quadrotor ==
function [m,J,r_oc] = add_load(m_0,J_0,r_oc_0,m_l,J_l,r_ol)
%#codegen
r_oc = (m_0*r_oc_0 + m_l*r_ol)/(m_0+m_l); 
m = m_0 + m_l; 
r_cl = -r_oc + r_ol; 
r_co = -r_oc; 
J = J_0 + J_l + m_0*(r_co'*r_co*eye(3) - r_co*r_co') + m_l*(r_cl'*r_cl*eye(3) - r_cl*r_cl'); 

end

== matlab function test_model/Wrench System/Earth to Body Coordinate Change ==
function x_B = earth2body(x_E,Theta)
%#codegen

phi = Theta(1); 
theta = Theta(2); 
psi = Theta(3); 

             
L_EB = [                           cos(theta)*cos(psi) ,                            cos(theta)*sin(psi) ,         -sin(theta) ; 
        sin(phi)*sin(theta)*cos(psi)-cos(phi)*sin(psi) , sin(phi)*sin(theta)*sin(psi)+cos(phi)*cos(psi) , sin(phi)*cos(theta) ; 
        cos(phi)*sin(theta)*cos(psi)+sin(phi)*sin(psi) , cos(phi)*sin(theta)*sin(psi)-sin(phi)*cos(psi) , cos(phi)*cos(theta)]; 

x_B = L_EB*x_E;  

end

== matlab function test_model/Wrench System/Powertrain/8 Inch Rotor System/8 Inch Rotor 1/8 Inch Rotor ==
function [F,Q] = rotor_8_inch(omega,alpha,v,Omega,K_T,K_H,K_d,r_h,Delta_T,Gamma_T,Gamma_H,Gamma_Omega,J_r)
%#codegen

% calculate hub velocity
v_h = v + cross(Omega,r_h); 

% calculate thrust
T = K_T*(omega^2)*Gamma_T;
% calculate H force
H = -K_H*omega*Gamma_H*v_h; %[-v(1);-v(2);-0.5*v(3)];

% calculate total force
F = T + H; 

% calculate force lever-arm torque 
Q_F = cross(r_h,F); 
% calculate drag torque 
Q_d = -K_d*(omega^2)*Gamma_Omega; 
% calculate gyroscopic torque 
Q_g = -cross( J_r*Omega, omega*Gamma_Omega ); 
% calculate in plane acceleration torque
Q_a = -J_r*alpha*Gamma_Omega; 
% produce torque vector
Q = Q_F + Q_d + Q_g + Q_a; 

end

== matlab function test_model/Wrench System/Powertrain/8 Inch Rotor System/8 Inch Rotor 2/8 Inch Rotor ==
function [F,Q] = rotor_8_inch(omega,alpha,v,Omega,K_T,K_H,K_d,r_h,Delta_T,Gamma_T,Gamma_H,Gamma_Omega,J_r)
%#codegen

% calculate hub velocity
v_h = v + cross(Omega,r_h); 

% calculate thrust
T = K_T*(omega^2)*Gamma_T;
% calculate H force
H = -K_H*omega*Gamma_H*v_h; %[-v(1);-v(2);-0.5*v(3)];

% calculate total force
F = T + H; 

% calculate force lever-arm torque 
Q_F = cross(r_h,F); 
% calculate drag torque 
Q_d = -K_d*(omega^2)*Gamma_Omega; 
% calculate gyroscopic torque 
Q_g = -cross( J_r*Omega, omega*Gamma_Omega ); 
% calculate in plane acceleration torque
Q_a = -J_r*alpha*Gamma_Omega; 
% produce torque vector
Q = Q_F + Q_d + Q_g + Q_a; 

end

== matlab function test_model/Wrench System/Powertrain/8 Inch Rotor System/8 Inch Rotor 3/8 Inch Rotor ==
function [F,Q] = rotor_8_inch(omega,alpha,v,Omega,K_T,K_H,K_d,r_h,Delta_T,Gamma_T,Gamma_H,Gamma_Omega,J_r)
%#codegen

% calculate hub velocity
v_h = v + cross(Omega,r_h); 

% calculate thrust
T = K_T*(omega^2)*Gamma_T;
% calculate H force
H = -K_H*omega*Gamma_H*v_h; %[-v(1);-v(2);-0.5*v(3)];

% calculate total force
F = T + H; 

% calculate force lever-arm torque 
Q_F = cross(r_h,F); 
% calculate drag torque 
Q_d = -K_d*(omega^2)*Gamma_Omega; 
% calculate gyroscopic torque 
Q_g = -cross( J_r*Omega, omega*Gamma_Omega ); 
% calculate in plane acceleration torque
Q_a = -J_r*alpha*Gamma_Omega; 
% produce torque vector
Q = Q_F + Q_d + Q_g + Q_a; 

end

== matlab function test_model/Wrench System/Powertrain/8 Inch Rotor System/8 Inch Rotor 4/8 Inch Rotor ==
function [F,Q] = rotor_8_inch(omega,alpha,v,Omega,K_T,K_H,K_d,r_h,Delta_T,Gamma_T,Gamma_H,Gamma_Omega,J_r)
%#codegen

% calculate hub velocity
v_h = v + cross(Omega,r_h); 

% calculate thrust
T = K_T*(omega^2)*Gamma_T;
% calculate H force
H = -K_H*omega*Gamma_H*v_h; %[-v(1);-v(2);-0.5*v(3)];

% calculate total force
F = T + H; 

% calculate force lever-arm torque 
Q_F = cross(r_h,F); 
% calculate drag torque 
Q_d = -K_d*(omega^2)*Gamma_Omega; 
% calculate gyroscopic torque 
Q_g = -cross( J_r*Omega, omega*Gamma_Omega ); 
% calculate in plane acceleration torque
Q_a = -J_r*alpha*Gamma_Omega; 
% produce torque vector
Q = Q_F + Q_d + Q_g + Q_a; 

end

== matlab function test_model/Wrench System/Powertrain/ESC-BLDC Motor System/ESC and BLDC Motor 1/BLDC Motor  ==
function alpha = BLDC_motor(V,omega,R_m,K_Q,K_V,i_0,K_d,J_r)
%#codegen
alpha = 1/J_r*(V/(R_m*K_Q)-omega/(R_m*K_Q*K_V)-sign(omega)*i_0/K_Q-K_d*omega^2);
end

== matlab function test_model/Wrench System/Powertrain/ESC-BLDC Motor System/ESC and BLDC Motor 1/BLDC Motor 
(no transient) ==
function [alpha,omega] = BLDC_motor_no_transient(V,R_m,K_Q,K_V,i_0,K_d)
%#codegen
alpha = 0;
omega = (-1 + sqrt(1-4*R_m*K_d*K_Q*K_V*(K_V*R_m*i_0-K_V*V)))/(2*R_m*K_d*K_Q*K_V); 
% omega = 50.7815*(V-6.749)+470.0908; 
end

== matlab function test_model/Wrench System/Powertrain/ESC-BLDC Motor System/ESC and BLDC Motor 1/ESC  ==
function V = esc_cmd(p,V_b,K_E,p_0,p_max)
%#codegen

u_p = (p - p_0)/(p_max - p_0);

V = K_E*u_p*V_b; 

end

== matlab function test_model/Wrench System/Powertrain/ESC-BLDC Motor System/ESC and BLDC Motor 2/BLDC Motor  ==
function alpha = BLDC_motor(V,omega,R_m,K_Q,K_V,i_0,K_d,J_r)
%#codegen
alpha = 1/J_r*(V/(R_m*K_Q)-omega/(R_m*K_Q*K_V)-sign(omega)*i_0/K_Q-K_d*omega^2);
end

== matlab function test_model/Wrench System/Powertrain/ESC-BLDC Motor System/ESC and BLDC Motor 2/BLDC Motor 
(no transient) ==
function [alpha,omega] = BLDC_motor_no_transient(V,R_m,K_Q,K_V,i_0,K_d)
%#codegen
alpha = 0;
omega = (-1 + sqrt(1-4*R_m*K_d*K_Q*K_V*(K_V*R_m*i_0-K_V*V)))/(2*R_m*K_d*K_Q*K_V); 
% omega = 50.7815*(V-6.749)+470.0908; 
end

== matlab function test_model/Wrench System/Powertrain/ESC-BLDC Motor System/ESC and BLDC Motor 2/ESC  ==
function V = esc_cmd(p,V_b,K_E,p_0,p_max)
%#codegen

u_p = (p - p_0)/(p_max - p_0);

V = K_E*u_p*V_b; 

end

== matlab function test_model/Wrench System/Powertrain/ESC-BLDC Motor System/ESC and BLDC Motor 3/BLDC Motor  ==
function alpha = BLDC_motor(V,omega,R_m,K_Q,K_V,i_0,K_d,J_r)
%#codegen
alpha = 1/J_r*(V/(R_m*K_Q)-omega/(R_m*K_Q*K_V)-sign(omega)*i_0/K_Q-K_d*omega^2);
end

== matlab function test_model/Wrench System/Powertrain/ESC-BLDC Motor System/ESC and BLDC Motor 3/BLDC Motor 
(no transient) ==
function [alpha,omega] = BLDC_motor_no_transient(V,R_m,K_Q,K_V,i_0,K_d)
%#codegen
alpha = 0;
omega = (-1 + sqrt(1-4*R_m*K_d*K_Q*K_V*(K_V*R_m*i_0-K_V*V)))/(2*R_m*K_d*K_Q*K_V); 
% omega = 50.7815*(V-6.749)+470.0908; 
end

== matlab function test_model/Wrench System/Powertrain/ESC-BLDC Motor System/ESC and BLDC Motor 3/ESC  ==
function V = esc_cmd(p,V_b,K_E,p_0,p_max)
%#codegen

u_p = (p - p_0)/(p_max - p_0);

V = K_E*u_p*V_b; 

end

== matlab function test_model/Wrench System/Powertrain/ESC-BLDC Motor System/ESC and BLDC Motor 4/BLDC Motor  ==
function alpha = BLDC_motor(V,omega,R_m,K_Q,K_V,i_0,K_d,J_r)
%#codegen
alpha = 1/J_r*(V/(R_m*K_Q)-omega/(R_m*K_Q*K_V)-sign(omega)*i_0/K_Q-K_d*omega^2);
end

== matlab function test_model/Wrench System/Powertrain/ESC-BLDC Motor System/ESC and BLDC Motor 4/BLDC Motor 
(no transient) ==
function [alpha,omega] = BLDC_motor_no_transient(V,R_m,K_Q,K_V,i_0,K_d)
%#codegen
alpha = 0;
omega = (-1 + sqrt(1-4*R_m*K_d*K_Q*K_V*(K_V*R_m*i_0-K_V*V)))/(2*R_m*K_d*K_Q*K_V); 
% omega = 50.7815*(V-6.749)+470.0908; 
end

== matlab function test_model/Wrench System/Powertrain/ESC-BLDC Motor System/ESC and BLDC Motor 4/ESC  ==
function V = esc_cmd(p,V_b,K_E,p_0,p_max)
%#codegen

u_p = (p - p_0)/(p_max - p_0);

V = K_E*u_p*V_b; 

end
